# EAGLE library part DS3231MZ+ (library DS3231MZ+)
Real Time Clock 5+/-ppm RTC Source: Datasheet
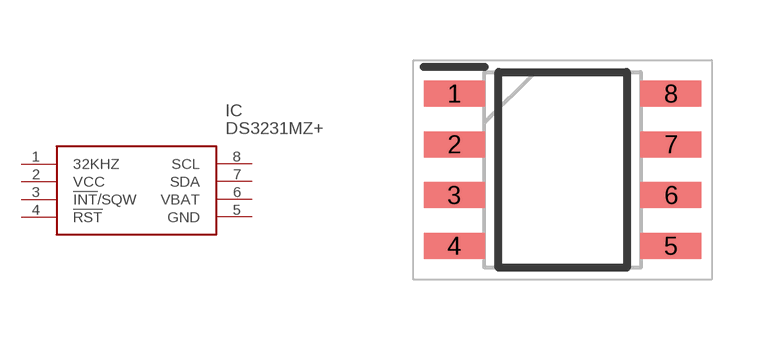
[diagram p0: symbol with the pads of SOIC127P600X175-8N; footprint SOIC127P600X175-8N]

Designator prefix IC

## DS3231MZ+ (Description: Real Time Clock 5+/-ppm RTC; Height: 1.75mm; Manufacturer_Name: Analog Devices; Manufacturer_Part_Number: DS3231MZ+; Mouser_Part_Number: 700-DS3231MZ+; Mouser_Price-Stock: https://www.mouser.co.uk/ProductDetail/Analog-Devices-Maxim-Integrated/DS3231MZ%2b?qs=4Rc5iGDDRGgASPOHxzykqQ%3D%3D)  [SOIC127P600X175-8N]
1  32KHZ
2  VCC
3  !INT!/SQW
4  !RST
5  GND
6  VBAT
7  SDA
8  SCL

## Footprint SOIC127P600X175-8N (pad centres in mm)
8 SO-3
smd 1.525 x 0.65: 1 -2.712,1.905; 2 -2.712,0.635; 3 -2.712,-0.635; 4 -2.712,-1.905; 5 2.712,-1.905; 6 2.712,-0.635; 7 2.712,0.635; 8 2.712,1.905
